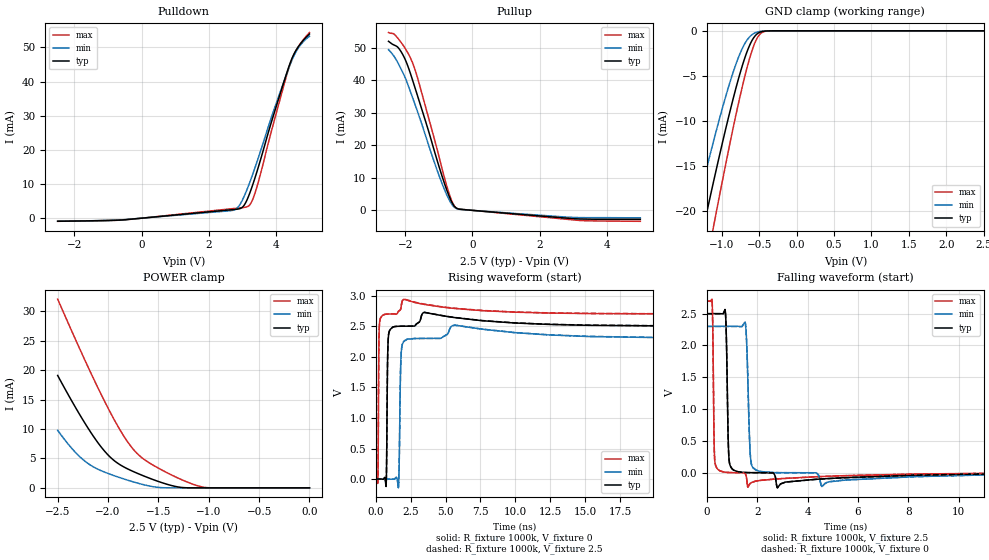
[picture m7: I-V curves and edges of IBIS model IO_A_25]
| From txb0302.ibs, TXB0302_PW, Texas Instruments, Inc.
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[Model]   IO_A_25
Model_type  3-state
Enable   Active-High
Vref =   0
Rref =   1000k
Cref =   50p
Vmeas =   1.25
| variable   typ   min   max
C_comp   3.26pF   3.05pF   3.41pF
| C_pullup   3.51pF   3.18pF   3.69pF
| C_pulldown   3.51pF   3.18pF   3.68pF
| C_tri-state   3.26pF   3.05pF   3.41pF
[Temperature Range]   40   100   -40
| Ambient temperature   25   85   -40
[Voltage range]   2.5   2.3   2.7
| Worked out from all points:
|   slope of the pulldown table from 0 to 0.375 V, typ, clamps not added: 1.08 kohm
|   slope of the pullup table from 0 to 0.375 V, typ, clamps not added: 1.17 kohm
|   GND clamp passes 1 mA (typ) near -0.59 V on its own axis
|   POWER clamp passes 1 mA (typ) near -1.49 V on its own axis
|   rising waveform, R_fixture 1000k, V_fixture 0: 20-80 % time 64.9ps typ, 91.1ps min, 44.1ps max; typ from 0 V to 2.5 V
|   falling waveform, R_fixture 1000k, V_fixture 2.5: 20-80 % time 67.4ps typ, 101ps min, 46.5ps max; typ from 2.5 V to 0.003 V
|   rising waveform, R_fixture 1000k, V_fixture 2.5: 20-80 % time 65.1ps typ, 91ps min, 44.1ps max; typ from 0.003 V to 2.5 V
|   falling waveform, R_fixture 1000k, V_fixture 0: 20-80 % time 67.3ps typ, 101ps min, 46.6ps max; typ from 2.5 V to 0 V
[GND Clamp]
| IO_A_25
|   Voltage   I(typ)   I(min)   I(max)
-2.5V     -73.32mA   -63.17mA   -85.42mA
-1.405V   -28.12mA   -22.26mA   -34.82mA
-1.37V    -26.74mA   -21.03mA   -33.25mA
-1.23V    -21.32mA   -16.24mA   -27.03mA
-1.11V    -16.79mA   -12.29mA   -21.77mA
-940mV    -10.66mA   -7.1mA     -14.54mA
-790mV    -5.749mA   -3.248mA   -8.575mA
-665mV    -2.391mA   -1.068mA   -4.201mA
-565mV    -678.3uA   -271.2uA   -1.498mA
-490mV    -156.8uA   -67.87uA   -382.1uA
-385mV    -10.8uA    -5.431uA   -18.51uA
2.5V      503.5pA    182.5nA    46.46pA
[POWER Clamp]
| IO_A_25
|   Voltage   I(typ)   I(min)   I(max)
-2.5V     19.09mA    9.777mA    32.05mA
-2.375V   15.21mA    7.012mA    27.2mA
-2.265V   11.98mA    5.048mA    23.01mA
-2.16V    9.134mA    3.71mA     19.13mA
-2.035V   6.25mA     2.679mA    14.73mA
-1.935V   4.576mA    2.042mA    11.46mA
-1.82V    3.346mA    1.386mA    8.173mA
-1.735V   2.666mA    944.4uA    6.274mA
-1.65V    2.054mA    551.9uA    4.94mA
-1.325V   220uA      589.8nA    1.823mA
-1.05V    66.45nA    29.78nA    108uA
0V        0A         0A         0A
[Pulldown]
| IO_A_25
|   Voltage   I(typ)   I(min)   I(max)
-2.5V     -903.8uA   -889.2uA   -911.8uA
-525mV    -480.4uA   -436.1uA   -524.8uA
2.705V    2.498mA    2.275mA    2.793mA
2.855V    2.651mA    3.047mA    2.948mA
2.995V    3.148mA    5.176mA    3.093mA
3.185V    6.422mA    9.542mA    3.563mA
3.3V      9.522mA    12.61mA    5.307mA
3.44V     13.79mA    16.61mA    9.364mA
3.885V    28.77mA    30.11mA    26.19mA
4.43V     45.58mA    45.14mA    45.36mA
4.675V    50.33mA    49.95mA    50.35mA
5V        53.95mA    53.29mA    54.36mA
[Pullup]
| IO_A_25
|   Voltage   I(typ)   I(min)   I(max)
-2.5V     51.97mA    49.38mA    54.64mA
-2.33V    50.79mA    47.28mA    54.14mA
-2.115V   48.59mA    43.23mA    51.47mA
-1.955V   45.19mA    39.53mA    48.96mA
-1.77V    39.61mA    34.27mA    44.99mA
-1.565V   32.92mA    28.25mA    38.15mA
-1.155V   19mA       15.41mA    22.74mA
-890mV    10.03mA    7.86mA     12.22mA
-655mV    3.411mA    2.539mA    3.963mA
-490mV    779.7uA    631.7uA    794.7uA
3.19V     -2.641mA   -2.22mA    -3.098mA
5V        -2.76mA    -2.282mA   -3.359mA
[Ramp]
| IO_A_25
| variable   typ   min   max
dV/dt_r   1.71/8.77E-11   1.60/1.24E-10   1.80/5.82E-11
dV/dt_f   1.68/8.37E-11   1.55/1.32E-10   1.77/5.79E-11
R_load = 1000k
[Rising Waveform]
| IO_A_25
R_fixture =   1000k
C_fixture =   0
L_fixture =   0
V_fixture =   0
V_fixture_min = 0
V_fixture_max = 0
|   Time   V(typ)   V(min)   V(max)
0s        551.5nV    2.547uV    74.85nV
141ps     7.176uV    2.544uV    -39.11mV
213ps     -45.98uV   2.563uV    2.197V
277ps     -90.78uV   2.565uV    2.586V
733ps     -119.5mV   10.87uV    2.695V
909ps     2.361V     -108.1uV   2.698V
1.613ns   2.498V     -141.7mV   2.742V
1.781ns   2.499V     1.887V     2.786V
1.981ns   2.499V     2.245V     2.936V
37.53ns   2.497V     2.297V     2.697V
[Falling Waveform]
| IO_A_25
R_fixture =   1000k
C_fixture =   0
L_fixture =   0
V_fixture =   2.5
V_fixture_min = 2.3
V_fixture_max = 2.7
|   Time   V(typ)   V(min)   V(max)
0s        2.5V       2.3V       2.7V
213ps     2.5V       2.3V       2.703V
333ps     2.5V       2.3V       143.6mV
733ps     2.552V     2.3V       8.201mV
909ps     138.1mV    2.3V       3.309mV
1.525ns   3.54mV     2.366V     -12.34mV
1.629ns   2.273mV    1.49V      -225.5mV
1.829ns   1.071mV    81.71mV    -145.9mV
4.565ns   -97.25mV   -217.5mV   -59.26mV
37.53ns   2.721mV    2.985mV    2.611mV
[Rising Waveform]
| IO_A_25
R_fixture =   1000k
C_fixture =   0
L_fixture =   0
V_fixture =   2.5
V_fixture_min = 2.3
V_fixture_max = 2.7
|   Time   V(typ)   V(min)   V(max)
0s        2.683mV    2.747mV    2.604mV
141ps     2.69mV     2.747mV    -36.57mV
213ps     2.637mV    2.747mV    2.198V
277ps     2.592mV    2.747mV    2.586V
733ps     -116.8mV   2.756mV    2.695V
909ps     2.362V     2.638mV    2.698V
1.613ns   2.498V     -139.1mV   2.743V
1.781ns   2.499V     1.887V     2.785V
2.005ns   2.499V     2.251V     2.942V
37.53ns   2.5V       2.3V       2.7V
[Falling Waveform]
| IO_A_25
R_fixture =   1000k
C_fixture =   0
L_fixture =   0
V_fixture =   0
V_fixture_min = 0
V_fixture_max = 0
|   Time   V(typ)   V(min)   V(max)
0s        2.497V     2.297V     2.697V
213ps     2.497V     2.297V     2.701V
333ps     2.497V     2.297V     143.4mV
733ps     2.55V      2.297V     8.139mV
901ps     154.5mV    2.297V     3.382mV
1.525ns   3.486mV    2.363V     -12.36mV
1.629ns   2.218mV    1.487V     -226.2mV
1.829ns   1.017mV    81.54mV    -144.2mV
4.573ns   -98.15mV   -215.1mV   -59.75mV
37.53ns   40.17uV    248uV      8.114uV
